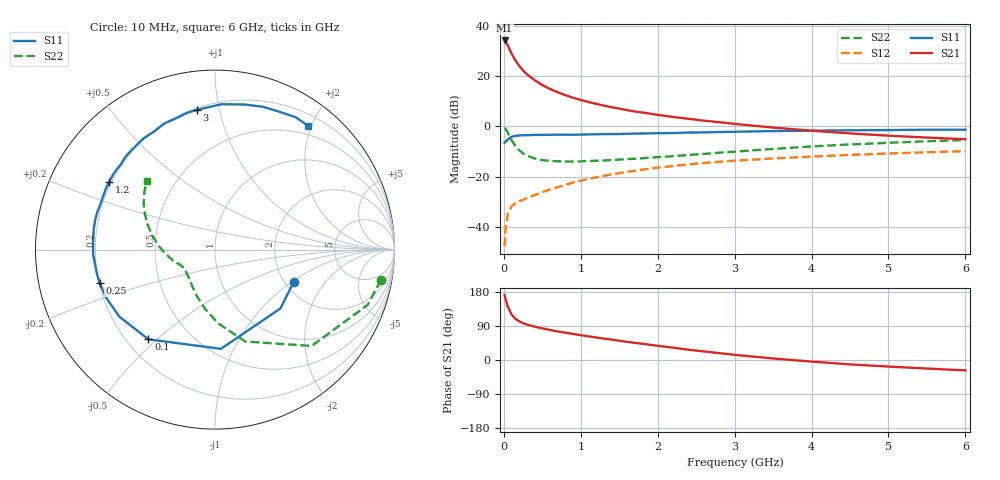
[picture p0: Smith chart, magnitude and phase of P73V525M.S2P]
! SIEMENS Small Signal Semiconductors
! BFP196
! Si NPN RF Bipolar Junction Transistor in SOT143
! VCE = 3.5 V  IC = 25 mA
! Common Emitter S-Parameters:  May  1996
# GHz  S  MA  R  50
!  f  S11  S21  S12  S22
! GHz  MAG  ANG  MAG  ANG  MAG  ANG  MAG  ANG
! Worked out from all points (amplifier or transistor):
!   36 points, 10 MHz to 6 GHz, reference 50 ohm
!   highest |S21| = 34.2 dB at 10 MHz (marker M1)
!   |S21| within 3 dB of that: start of sweep to 66.37 MHz
!   unconditionally stable (mu >= 1): 615.4 MHz to 3.492 GHz; 3.666 GHz to 4.019 GHz
!   at 250 MHz: K = 0.67, MSG = 25.7 dB, |S12| = -29.1 dB
!   at 1.4 GHz: K = 1.11, MAG = 11.4 dB, |S12| = -19.1 dB
!   at 6 GHz: K = 0.97, MSG = 2.4 dB, |S12| = -9.8 dB
!   S11 on the Smith chart (normalised r, x): 10 MHz: 2.24, -1.03; 100 MHz: 0.29, -0.47; 250 MHz: 0.20, -0.13; 1.2 GHz: 0.19, +0.28; 3 GHz: 0.21, +0.86; 6 GHz: 0.36, +1.95
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0.01  0.4745 -22.0  51.09 171.4  0.0042 83.2  0.9401 -10.4
0.02  0.4902 -42.0  48.83 162.0  0.0085 75.4  0.9045 -19.9
0.05  0.554 -86.6  40.84 141.2  0.0181 59.6  0.7606 -44.9
0.1  0.6226 -126.6  28.18 120.2  0.026 46.0  0.5388 -71.8
0.15  0.6509 -145.0  20.51 108.9  0.0298 42.6  0.4111 -87.6
0.2  0.6631 -156.2  16.02 102.0  0.0326 42.7  0.338 -98.9
0.25  0.6693 -164.0  12.94 97.1  0.035 44.0  0.2917 -107.9
0.3  0.6717 -169.0  10.91 93.6  0.0378 46.3  0.2657 -114.5
0.4  0.6799 -178.0  8.304 88.1  0.0434 49.0  0.2317 -124.9
0.5  0.6798 176.4  6.655 83.5  0.0497 51.5  0.215 -132.6
0.6  0.6849 170.9  5.565 79.3  0.0561 53.2  0.2071 -138.0
0.7  0.6875 166.2  4.785 75.3  0.0624 54.6  0.2037 -142.2
0.9  0.6867 158.6  3.727 68.8  0.077 55.2  0.201 -148.4
1.1  0.6963 151.0  3.064 62.5  0.0906 55.1  0.2061 -152.5
1.2  0.7004 147.3  2.813 59.5  0.0976 54.8  0.2088 -154.6
1.6  0.717 134.5  2.113 48.0  0.1256 51.3  0.2253 -160.9
2.2  0.7405 117.2  1.545 32.5  0.1643 44.5  0.2573 -170.1
3  0.7852 97.3  1.126 13.6  0.2096 34.1  0.3166 175.7
3.5  0.8106 87.5  0.952 4.1  0.2321 27.7  0.3584 167.2
4.5  0.8399 71.3  0.729 -11.6  0.2726 16.1  0.4394 152.8
5.5  0.8638 58.7  0.602 -22.6  0.3079 5.4  0.5086 140.7
6  0.8629 53.1  0.559 -27.4  0.3243 -0.4  0.5393 134.8
